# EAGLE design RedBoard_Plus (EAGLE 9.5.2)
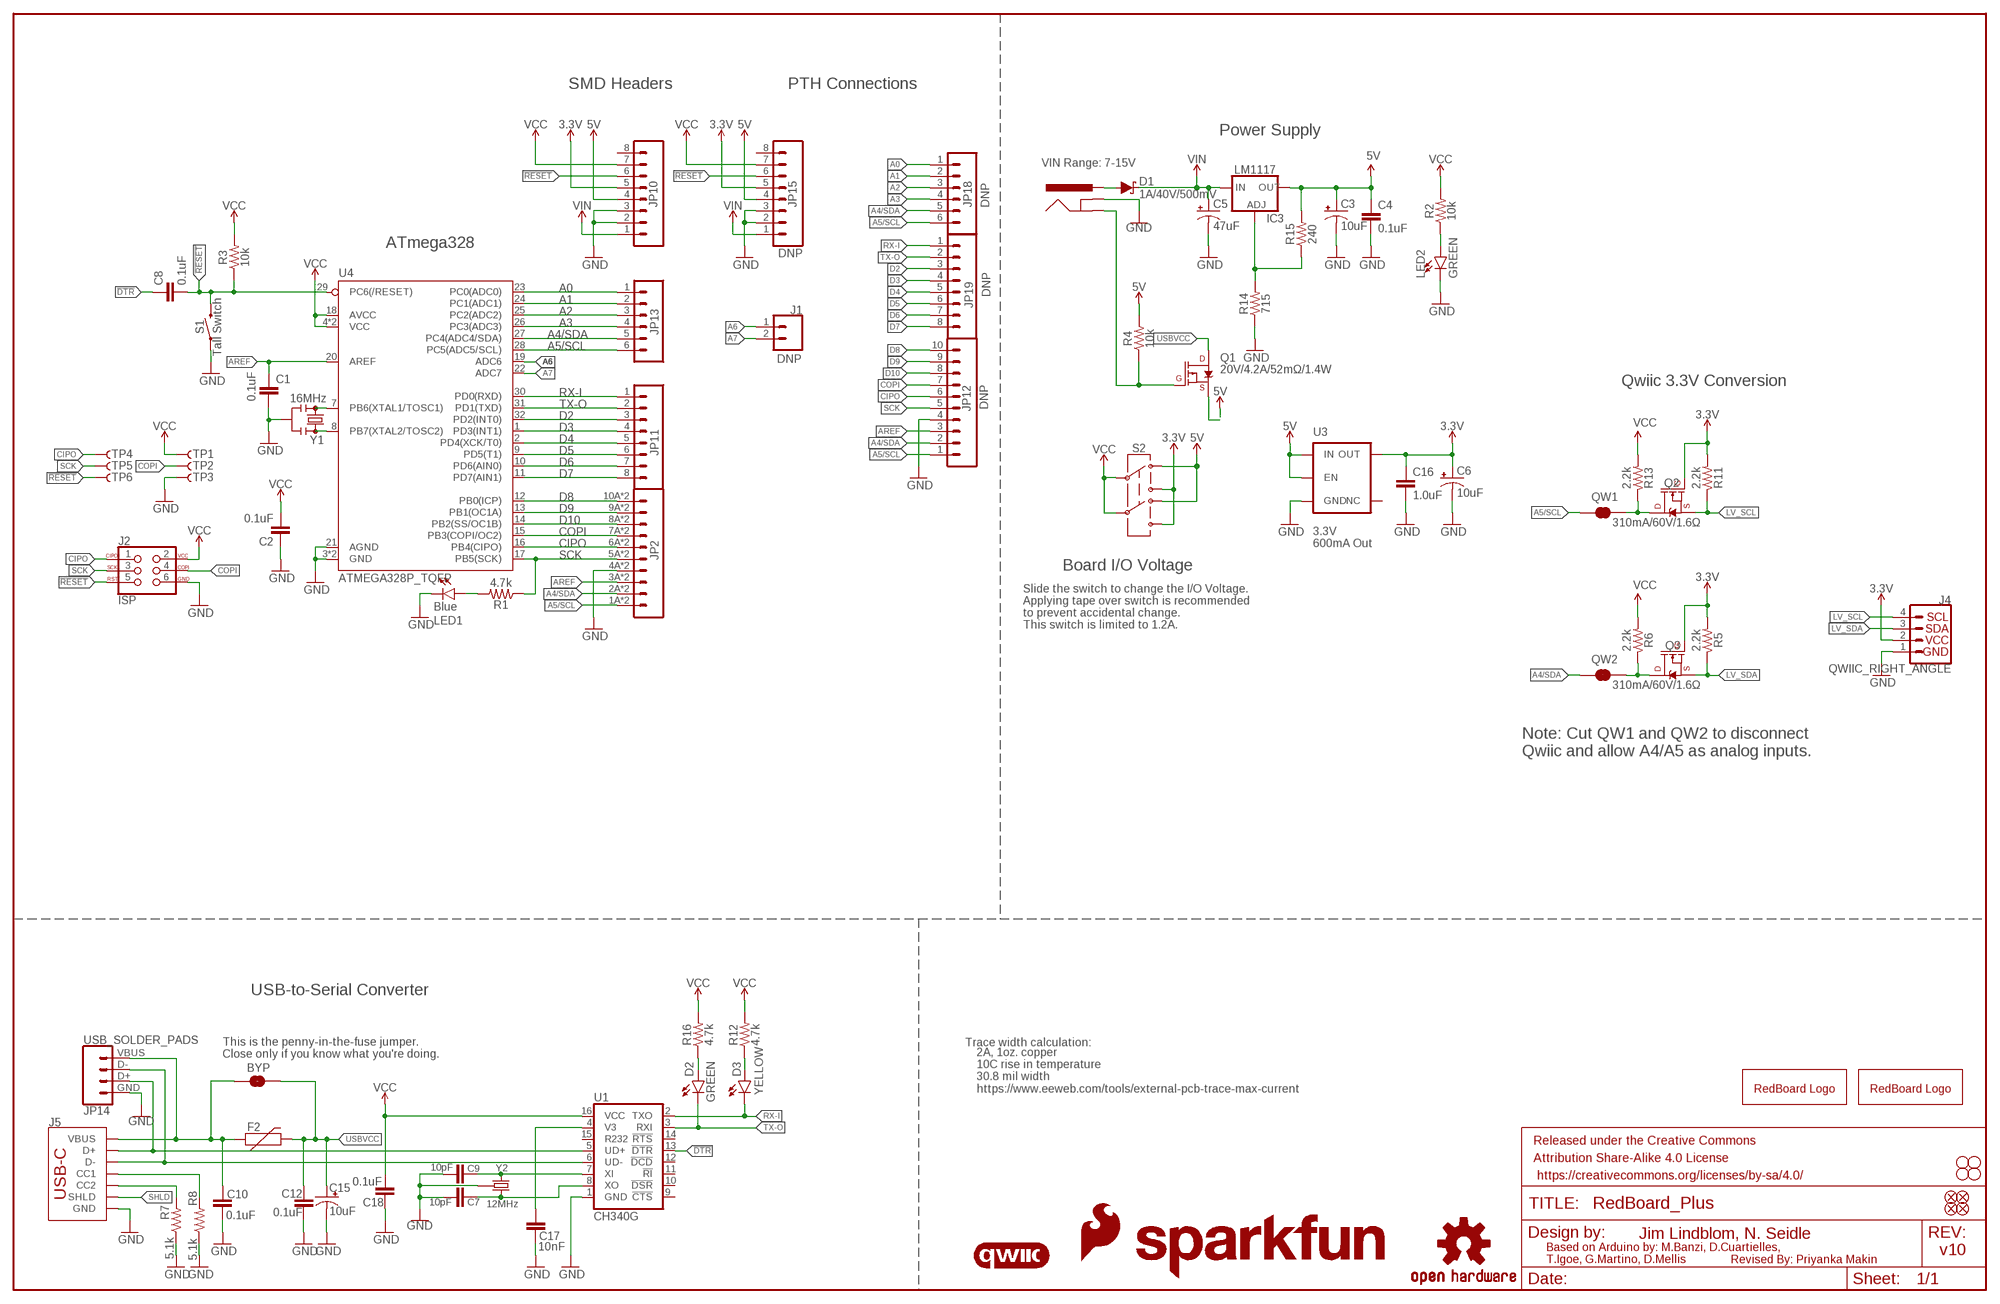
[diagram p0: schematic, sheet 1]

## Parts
BYP  JUMPER-SMT_2_NO_SILK  [SMT-JUMPER_2_NO_SILK]
C1  0.1uF  0.1UF-0603-25V-(+80/-20%)  [0603]
C2  0.1uF  0.1UF-0603-25V-(+80/-20%)  [0603]
C3  10uF  10UF-POLAR-EIA3216-16V-10%(TANT)  [EIA3216]
C4  0.1uF  0.1UF-0603-25V-(+80/-20%)  [0603]
C5  47uF  47UF-POLAR-PANASONIC_D-35V-20%  [PANASONIC_D]
C6  10uF  10UF-POLAR-EIA3216-16V-10%(TANT)  [EIA3216]
C7  10pF  10PF-0603-50V-5%  [0603]
C8  0.1uF  0.1UF-0603-25V-(+80/-20%)  [0603]
C9  10pF  10PF-0603-50V-5%  [0603]
C10  0.1uF  0.1UF-0603-25V-(+80/-20%)  [0603]
C12  0.1uF  0.1UF-0603-25V-(+80/-20%)  [0603]
C15  10uF  10UF-POLAR-EIA3216-16V-10%(TANT)  [EIA3216]
C16  1.0uF  1.0UF-0603-16V-10%  [0603]
C17  10nF  10NF-0603-50V-10%  [0603]
C18  0.1uF  0.1UF-0603-25V-(+80/-20%)  [0603]
D1  1A/40V/500mV  DIODE-SCHOTTKY-SS14  [SMA-DIODE]
D2  GREEN  LED-GREENLILYPAD  [LED-1206]
D3  YELLOW  LED-YELLOW_HIDDENSILK  [LED-1206-HIDDENSILK]
F2  6V/2A  PPTC_6V2A  [1210]
FD1  FIDUCIAL1X2  [FIDUCIAL-1X2]
FD2  FIDUCIAL1X2  [FIDUCIAL-1X2]
FRAME1  FRAME-LEDGER  [CREATIVE_COMMONS]
IC3  LM1117  V_REG_LM1117SOT223  [SOT223]
J1  DNP  CONN_021X02_NO_SILK  [1X02_NO_SILK]
J2  ISP  AVR_SPI_PROG_3X2SMD  [2X3_SMT_POSTS]
J3  5.5x2.1mm Barrel  POWER_JACKSMD  [POWER_JACK_SMD]
J4  QWIIC_RIGHT_ANGLE  QWIIC_CONNECTORJS-1MM  [JST04_1MM_RA]
J5  USB Female Type C Connector  USB_C_2-LAYER_PADS  [USB-C-16P-2LAYER-PADS]
JP1  SFE_LOGO_NAME.1_INCH  [SFE_LOGO_NAME_.1]
JP2  CONN_10SMD_COMBO-FEMALE  [1X10_SMD_COMBINED]
JP3  STAND-OFFTIGHT  [STAND-OFF-TIGHT]
JP4  STAND-OFFTIGHT  [STAND-OFF-TIGHT]
JP5  STAND-OFFTIGHT  [STAND-OFF-TIGHT]
JP6  STAND-OFFTIGHT  [STAND-OFF-TIGHT]
JP7  SFE_LOGO_FLAME.1_INCH  [SFE_LOGO_FLAME_.1]
JP8  FIDUCIAL1X2  [FIDUCIAL-1X2]
JP9  FIDUCIAL1X2  [FIDUCIAL-1X2]
JP10  CONN_08SMD-COMBO-FEMALE  [1X08_SMD_COMBINED]
JP11  JP11  CONN_08SMD-COMBO-FEMALE  [1X08_SMD_COMBINED]
JP12  DNP  CONN_10NO_SILK_PTH_FEMALE  [1X10_NO_SILK]
JP13  CONN_06SMD-STRAIGHT-COMBO-FEMALE  [1X06_SMD_STRAIGHT_COMBO]
JP14  USB_SOLDER_PADS  [USB-SOLDER-PADS]
JP15  DNP  CONN_08NO_SILK_DNP  [1X08_NO_SILK]
JP18  DNP  CONN_06NO_SILK_NO_POP  [1X06_NO_SILK]
JP19  DNP  CONN_08NO_SILK_DNP  [1X08_NO_SILK]
LED1  Blue  LED-BLUE_HIDDENSILK  [LED-1206-HIDDENSILK]
LED2  GREEN  LED-GREENLILYPAD  [LED-1206]
LOGO1  QWIIC_LOGO_5MM  [QWIIC_5MM]
Q1  20V/4.2A/52mΩ/1.4W  MOSFET_PCH-DMG2305UX-7  [SOT23-3]
Q2  310mA/60V/1.6Ω  MOSFET-NCH-2N7002PW  [SOT323]
Q3  310mA/60V/1.6Ω  MOSFET-NCH-2N7002PW  [SOT323]
QW1  JUMPER-SMT_2_NC_TRACE_SILK  [SMT-JUMPER_2_NC_TRACE_SILK]
QW2  JUMPER-SMT_2_NC_TRACE_SILK  [SMT-JUMPER_2_NC_TRACE_SILK]
R1  4.7k  4.7KOHM-0603-1/10W-1%  [0603]
R2  10k  10KOHM-0603-1/10W-1%  [0603]
R3  10k  10KOHM-0603-1/10W-1%  [0603]
R4  10k  10KOHM-0603-1/10W-1%  [0603]
R5  2.2k  2.2KOHM-0603-1/10W-1%  [0603]
R6  2.2k  2.2KOHM-0603-1/10W-1%  [0603]
R7  5.1k  5.1KOHM5.1KOHM-0603-1/10W-1%  [0603]
R8  5.1k  5.1KOHM5.1KOHM-0603-1/10W-1%  [0603]
R11  2.2k  2.2KOHM-0603-1/10W-1%  [0603]
R12  4.7k  4.7KOHM-0603-1/10W-1%  [0603]
R13  2.2k  2.2KOHM-0603-1/10W-1%  [0603]
R14  715  715OHM-0603-1/10W-1%  [0603]
R15  240  240OHM-0603-1/10W-1%  [0603]
R16  4.7k  4.7KOHM-0603-1/10W-1%  [0603]
S1  Tall Switch  MOMENTARY-SWITCH-SPST-SMD-5.2-TALL-REDUNDANT  [TACTILE_SWITCH_SMD_5.2MM]
S2  SWITCH-DPDT-SMD-AYZ0202  [SWITCH_DPDT_SMD_AYZ0202]
TP1  TP-3x5  TEST-POINT3X5  [PAD.03X.05]
TP2  TP-3x5  TEST-POINT3X5  [PAD.03X.05]
TP3  TP-3x5  TEST-POINT3X5  [PAD.03X.05]
TP4  TP-3x5  TEST-POINT3X5  [PAD.03X.05]
TP5  TP-3x5  TEST-POINT3X5  [PAD.03X.05]
TP6  TP-3x5  TEST-POINT3X5  [PAD.03X.05]
U1  CH340G  CH340GSMD  [SO016]
U3  3.3V  V_REG_AP2112K-3.3V  [SOT23-5]
U4  ATMEGA328P_TQFP  [TQFP32-08]
U$1  REDBOARD_LOGO  [REDBOARD_LOGO]
U$3  REDBOARD_LOGO  [REDBOARD_LOGO]
U$16  OSHW-LOGOS  [OSHW-LOGO-S]
Y1  16MHz  RESONATOR-16MHZSMD_3.2X1.3  [RESONATOR-SMD-3.2X1.3]
Y2  12MHz  CRYSTAL-GROUNDEDSMD-3.2X2.5  [CRYSTAL-SMD-3.2X2.5MM]

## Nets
3.3V [power]: C6.+ C16.1 J4.2 JP10.5 JP15.5 Q2.1(G) Q3.1(G) R5.2 R11.2 S2.1 S2.4 U3.5(OUT)
5V [power]: C3.+ C4.1 IC3.2(OUT) IC3.4(OUT) JP10.4 JP15.4 Q1.2(S) R4.2 R15.2 S2.3 S2.6 U3.1(IN) U3.3(EN)
!DTR!: C8.1 U1.13(!DTR)
!RESET: C8.2 J2.5 JP10.6 JP15.6 R3.1 S1.3 S1.4 TP6.P$1 U4.29(PC6(/RESET))
A0: JP13.1 JP18.1 U4.23(PC0(ADC0))
A1: JP13.2 JP18.2 U4.24(PC1(ADC1))
A2: JP13.3 JP18.3 U4.25(PC2(ADC2))
A3: JP13.4 JP18.4 U4.26(PC3(ADC3))
A4/SDA: JP2.2A JP2.2B JP12.2 JP13.5 JP18.5 QW2.1 U4.27(PC4(ADC4/SDA))
A5/SCL: JP2.1A JP2.1B JP12.1 JP13.6 JP18.6 QW1.1 U4.28(PC5(ADC5/SCL))
A6: J1.1 U4.19(ADC6)
A7: J1.2 U4.22(ADC7)
AREF: C1.1 JP2.3A JP2.3B JP12.3 U4.20(AREF)
CC1: J5.A5(CC1) R8.2
CC2: J5.B5(CC2) R7.2
CIPO: J2.1 JP2.6A JP2.6B JP12.6 TP4.P$1 U4.16(PB4(CIPO))
COPI: J2.4 JP2.7A JP2.7B JP12.7 TP2.P$1 U4.15(PB3(COPI/OC2))
D2: JP11.3 JP19.3 U4.32(PD2(INT0))
D3: JP11.4 JP19.4 U4.1(PD3(INT1))
D4: JP11.5 JP19.5 U4.2(PD4(XCK/T0))
D5: JP11.6 JP19.6 U4.9(PD5(T1))
D6: JP11.7 JP19.7 U4.10(PD6(AIN0))
D7: JP11.8 JP19.8 U4.11(PD7(AIN1))
D8: JP2.10A JP2.10B JP12.10 U4.12(PB0(ICP))
D9: JP2.9A JP2.9B JP12.9 U4.13(PB1(OC1A))
D10: JP2.8A JP2.8B JP12.8 U4.14(PB2(SS/OC1B))
D+: J5.A6(D+) J5.B6(D+) JP14.D+ U1.5(UD+)
D-: J5.A7(D-) J5.B7(D-) JP14.D- U1.6(UD-)
GND: C1.2 C2.1 C3.- C4.2 C5.- C6.- C7.2 C9.2 C10.2 C12.2 C15.- C16.2 C17.2 C18.2 J2.6 J3.GND(GNDBREAK) J4.1 J5.GND J5.GND2(GND) JP2.4A JP2.4B JP10.2 JP10.3 JP12.4 JP14.GND JP15.2 JP15.3 LED1.C LED2.C R7.1 R8.1 R14.1 S1.1 S1.2 TP3.P$1 U1.1(GND) U3.2(GND) U4.3(GND) U4.5(GND) U4.21(AGND) Y1.2 Y2.2(GND) Y2.4(GND)
INSERT: J3.P$4(GND) Q1.1(G) R4.1
LV_SCL: J4.4 Q2.2(S) R11.1
LV_SDA: J4.3 Q3.2(S) R5.1
N$1: LED1.A R1.2
N$2: LED2.A R2.1
N$3: U4.7(PB6(XTAL1/TOSC1)) Y1.1
N$4: U4.8(PB7(XTAL2/TOSC2)) Y1.3
N$5: D2.A R16.1
N$6: C17.1 U1.4(V3)
N$7: Q2.3(D) QW1.2 R13.1
N$8: C9.1 U1.7(XI) Y2.1
N$9: D3.A R12.1
N$10: C7.1 U1.8(XO) Y2.3
N$15: IC3.1(ADJ) R14.2 R15.1
N$45: Q3.3(D) QW2.2 R6.1
PWRIN [power]: D1.A J3.VIN0(PWR)
RX-I: D3.C JP11.1 JP19.1 U1.2(TXO) U4.30(PD0(RXD))
SCK: J2.3 JP2.5A JP2.5B JP12.5 R1.1 TP5.P$1 U4.17(PB5(SCK))
SHLD: J5.SHLD1(SHLD) J5.SHLD2(SHLD) J5.SHLD3(SHLD) J5.SHLD4(SHLD)
TX-O: D2.C JP11.2 JP19.2 U1.3(RXI) U4.31(PD1(TXD))
USBVCC [power]: BYP.2 C12.1 C15.+ F2.2 Q1.3(D)
VCC: C2.2 C18.1 J2.2 JP10.7 JP15.7 R2.2 R3.2 R6.2 R12.2 R13.2 R16.2 S2.2 S2.5 TP1.P$1 U1.16(VCC) U4.4(VCC) U4.6(VCC) U4.18(AVCC)
VIN [power]: C5.+ D1.C IC3.3(IN) JP10.1 JP15.1
VUSB [power]: BYP.1 C10.1 F2.1 J5.VBUS1(VBUS) J5.VBUS2(VBUS) JP14.VBUS
Unconnected: JP10.8 JP15.8 U1.9(!CTS) U1.10(!DSR) U1.11(!RI) U1.12(!DCD) U1.14(!RTS) U1.15(R232) U3.4(NC)

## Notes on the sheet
- SMD Headers | PTH Connections
- Power Supply
- VIN Range: 7-15V
- ATmega328
- Qwiic 3.3V Conversion
- 3.3V
  600mA Out
- Board I/O Voltage
- Slide the switch to change the I/O Voltage.
  Applying tape over switch is recommended
  to prevent accidental change.
- This switch is limited to 1.2A.
- Note: Cut QW1 and QW2 to disconnect 
  Qwiic and allow A4/A5 as analog inputs.
- USB-to-Serial Converter
- Trace width calculation:
- This is the penny-in-the-fuse jumper.
  Close only if you know what you're doing.
- 2A, 1oz. copper
  10C rise in temperature
  30.8 mil width
  https://www.eeweb.com/tools/external-pcb-trace-max-current
- Jim Lindblom, N. Seidle
- v10
- Based on Arduino by: M.Banzi, D.Cuartielles, 
  T.Igoe, G.Martino, D.Mellis
- Revised By: Priyanka Makin

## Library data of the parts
BYP = SparkFun-Jumpers:JUMPER-SMT_2_NO: Normally open jumper
C1 C2 C4 C8 C10 C12 C18 = SparkFun-Capacitors:0.1UF: 0.1µF ceramic capacitors; PROD_ID: CAP-00810
C3 C6 C15 = SparkFun-Capacitors:10UF-POLAR: 10.0µF polarized capacitors; PROD_ID: CAP-00811
C5 = SparkFun-Capacitors:47UF-POLAR: 47µF polarized capacitors; PROD_ID: CAP-08478
C7 C9 = SparkFun-Capacitors:10PF: 10pF ceramic capacitors; PROD_ID: CAP-11812
C16 = SparkFun-Capacitors:1.0UF: 1µF ceramic capacitors; PROD_ID: CAP-00868
C17 = SparkFun-Capacitors:10NF: 0.01uF/10nF/10,000pF ceramic capacitors; PROD_ID: CAP-00867
D1 = SparkFun-DiscreteSemi:DIODE-SCHOTTKY: Schottky diode; PROD_ID: DIO-08053
D2 LED2 = SparkFun-LED:LED-GREEN: Green SMD LED; PROD_ID: DIO-09910
D3 = SparkFun-LED:LED-YELLOW: Yellow SMD LED; PROD_ID: DIO-09909
F2 = SparkFun-Fuses:PPTC: Resettable Fuse PPTC; PROD_ID: RES-14313
FD1 FD2 JP8 JP9 = SparkFun-Aesthetics:FIDUCIAL: Fiducial Alignment Points
FRAME1 = SparkFun-Aesthetics:FRAME-LEDGER: Schematic Frame - Ledger
IC3 = SparkFun-IC-Power:V_REG_LM1117: Voltage Regulator LM1117 Standard adjustable voltage regulator but in SMD form. Spark Fun Electronics SKU : COM-00595; PROD_ID: VREG-08170
J1 = SparkFun-Connectors:CONN_02: Multi connection point. Often used as Generic Header-pin footprint for 0.1 inch spaced/style header connections
J2 = SparkFun-Connectors:AVR_SPI_PROG_3X2: AVR ISP 6 Pin This is the reduced ISP connector for AVR programming. Common on Arduino. This footprint will take up less PCB space and can be used with a 10-pin to 6-pin adapter such as SKU: BOB-08508 **Special note about "TEST_POINT" package. The stop mask is on the top side, so if you want your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; PROD_ID: CONN-11415
J3 = SparkFun-Connectors:POWER_JACK: Power Jack Connector This is the standard 5.5mm barrel jack for power. The PTH is the most common, proven, reliable, footprint. The Slot footprint only works if the mill layer is transmitted to the PCB fab house so be warned. Here are the connectors we sell at SparkFun: DC Barrel Power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; PROD_ID: CONN-08106; SF_ID: PRT-12748
J4 = SparkFun-Connectors:QWIIC_CONNECTOR: SparkFun I2C Standard Qwiic Connector An SMD 1mm pitch JST connector makes it easy and quick (get it? Qwiic?) to connect I2C devices to each other. The Qwiic system enables fast and solderless connection between popular platforms and various sensors and actuators. We carry 200mm, 100mm, 50mm, and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; PROD_ID: CONN-13694
J5 = SparkFun-Connectors:USB_C: USB Type C 16Pin Connector Super Speed pins not available on the 16-pin purely SMD connector so this part is best for USB 2.0 implementations. D1 and D2 are tied together enabling D+/- no matter which way the cable is plugged into the connector. The two channel configuration pins (CC1/2) are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; PROD_ID: CONN-14122
JP1 = SparkFun-Aesthetics:SFE_LOGO_NAME: SparkFun Font Logo
JP2 JP12 = SparkFun-Connectors:CONN_10: Multi connection point. Often used as Generic Header-pin footprint for 0.1 inch spaced/style header connections On any of the 0.1 inch spaced packages, you can populate with these: Break Away Headers - Straight (PRT-00116) Break Away Male Headers - Right Angle (PRT-00553) Female Headers (PRT-00115)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; PROD_ID: CONN-11219
JP3-JP6 = SparkFun-Hardware:STAND-OFF: Stand Off
JP7 = SparkFun-Aesthetics:SFE_LOGO_FLAME: SparkFun Flame Logo
JP10 JP11 = SparkFun-Connectors:CONN_08: Multi connection point. Often used as Generic Header-pin footprint for 0.1 inch spaced/style header connections On any of the 0.1 inch spaced packages, you can populate with these: Break Away Headers - Straight (PRT-00116) Break Away Male Headers - Right Angle (PRT-00553) Female Headers (PRT-00115)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; PROD_ID: CONN-10204; SF_ID: PRT-11543
JP13 JP18 = SparkFun-Connectors:CONN_06: Multi connection point. Often used as Generic Header-pin footprint for 0.1 inch spaced/style header connections On any of the 0.1 inch spaced packages, you can populate with these: Break Away Headers - Straight (PRT-00116) Break Away Male Headers - Right Angle (PRT-00553) Female Headers (PRT-00115)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; PROD_ID: CONN-10203
JP14 = SparkFun-Connectors:USB_SOLDER_PADS: Solder pad access to USB pins. Helpful to expose on PCBs so user can attach external USB connector if necessary.
JP15 = SparkFun-Connectors:CONN_08: Multi connection point. Often used as Generic Header-pin footprint for 0.1 inch spaced/style header connections On any of the 0.1 inch spaced packages, you can populate with these: Break Away Headers - Straight (PRT-00116) Break Away Male Headers - Right Angle (PRT-00553) Female Headers (PRT-00115)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; PROD_ID: CONN-10204
JP19 = SparkFun-Connectors:CONN_08: Multi connection point. Often used as Generic Header-pin footprint for 0.1 inch spaced/style header connections On any of the 0.1 inch spaced packages, you can populate with these: Break Away Headers - Straight (PRT-00116) Break Away Male Headers - Right Angle (PRT-00553) Female Headers (PRT-00115)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
LED1 = SparkFun-LED:LED-BLUE: Blue SMD LED; PROD_ID: DIO-09911
LOGO1 = SparkFun-Aesthetics:QWIIC_LOGO: Qwiic Logos for placement on schematic and PCB. The 5.5mm silk logo is best for placing next to Qwiic connector.
Q1 = SparkFun-DiscreteSemi:MOSFET_PCH: P-channel MOSFETs Voltage controlled devices that allow control of high current outputs. SparkFun Products: SparkFun ESP32 Thing SparkFun ESP8266 Thing SparkFun Pi Servo HAT V2 DMG2305UX-7 (20V/4.2A/SOT23-3); PROD_ID: TRANS-14388
Q2 Q3 = SparkFun-DiscreteSemi:MOSFET-NCH: N-channel MOSFETs Voltage controlled devices that allow control of high current outputs. SparkFun Products: SparkFun OpenScale SparkFun Digital Sandbox SparkFun Monster Moto Shield SparkFun MOSFET Power Controller; PROD_ID: TRANS-11151
QW1 QW2 = SparkFun-Jumpers:JUMPER-SMT_2_NC_TRACE: Normally closed trace jumper
R1 R12 R16 = SparkFun-Resistors:4.7KOHM: 4.7kΩ resistor; PROD_ID: RES-07857
R2-R4 = SparkFun-Resistors:10KOHM: 10kΩ resistor; PROD_ID: RES-00824
R5 R6 R11 R13 = SparkFun-Resistors:2.2KOHM: 2.2kΩ resistor; PROD_ID: RES-08272
R7 R8 = SparkFun-Resistors:5.1KOHM; PROD_ID: RES-12083
R14 = SparkFun-Resistors:715OHM: 715Ω resistor; PROD_ID: RES-07850
R15 = SparkFun-Resistors:240OHM: 240Ω resistor; PROD_ID: RES-07849
S1 = SparkFun-Switches:MOMENTARY-SWITCH-SPST: Momentary Switch (Pushbutton) - SPST; PROD_ID: SWCH-14139
S2 = SparkFun-Switches:SWITCH-DPDT: Double-Pole, Double-Throw (DPDT) Switch Double-pole, double-throw switches. Variant Overview PTH-GPI-152-3013 Used on SparkFun Geiger Counter SMD-AY0202 Surface Mount DPDT Switch (COM-00597) Used on e.g. LilyPad Arduino USB - ATmega32U4 Board; PROD_ID: SWCH-08179; SF_SKU: COM-00597
TP1-TP6 = SparkFun-Connectors:TEST-POINT: SparkFun Test Points
U1 = SparkFun-IC-Comms:CH340G: A simple USB 2.0 to Serial IC.; PROD_ID: IC-13498
U3 = SparkFun-IC-Power:V_REG_AP2112: AP2112 - 600mA CMOS LDO Regulator w/ Enable The AP2112 is CMOS process low dropout linear regulator with enable function, the regulator delivers a guaranteed 600mA (min.) continuous load current. Features Output Voltage Accuracy: ±1.5% Output Current: 600mA (Min.) Foldback Short Current Protection: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; PROD_ID: VREG-12457
U4 = SparkFun-IC-Microcontroller:ATMEGA328P_TQFP: Popular 328P in QFP Storefront component: ATmega328 - TQFP (COM-13448) Datasheet SparkFun Products SparkFun RedBoard - Programmed with Arduino (DEV-12757) Arduino Pro Mini 328 - 5V/16MHz (DEV-11113) Arduino Pro Mini 328 - 3.3V/8MHz (DEV-11114) SparkFun OpenLog (DEV-13712) SparkFun MicroView - OLED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; PROD_ID: IC-09069
U$1 U$3 = SparkFun-Aesthetics:REDBOARD_LOGO
U$16 = SparkFun-Aesthetics:OSHW-LOGO: Open-Source Hardware (OSHW) Logo
Y1 = SparkFun-Clocks:RESONATOR-16MHZ: 16MHz Resonator Digikey Example Frequency: 16MHz Frequency Stability: &plusmn;0.3% Frequency Tolerance: &plusmn;0.5% Capacitance: 15pF SparkFun Products SparkFun OpenLog SparkFun MicroView - OLED Arduino Module; PROD_ID: XTAL-08900
Y2 = SparkFun-Clocks:CRYSTAL-GROUNDED: Crystals w/ Ground Pin (Generic) These are passive quartz crystals, which can be used as a clock source for a microcontroller. Crystal's are usually two-terminal devices. A third terminal may be optionally connected to ground, as recommended by the manufaturer.; PROD_ID: XTAL-13518

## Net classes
0 default: width 0 mm, drill 0 mm
1 power: width 0.762 mm

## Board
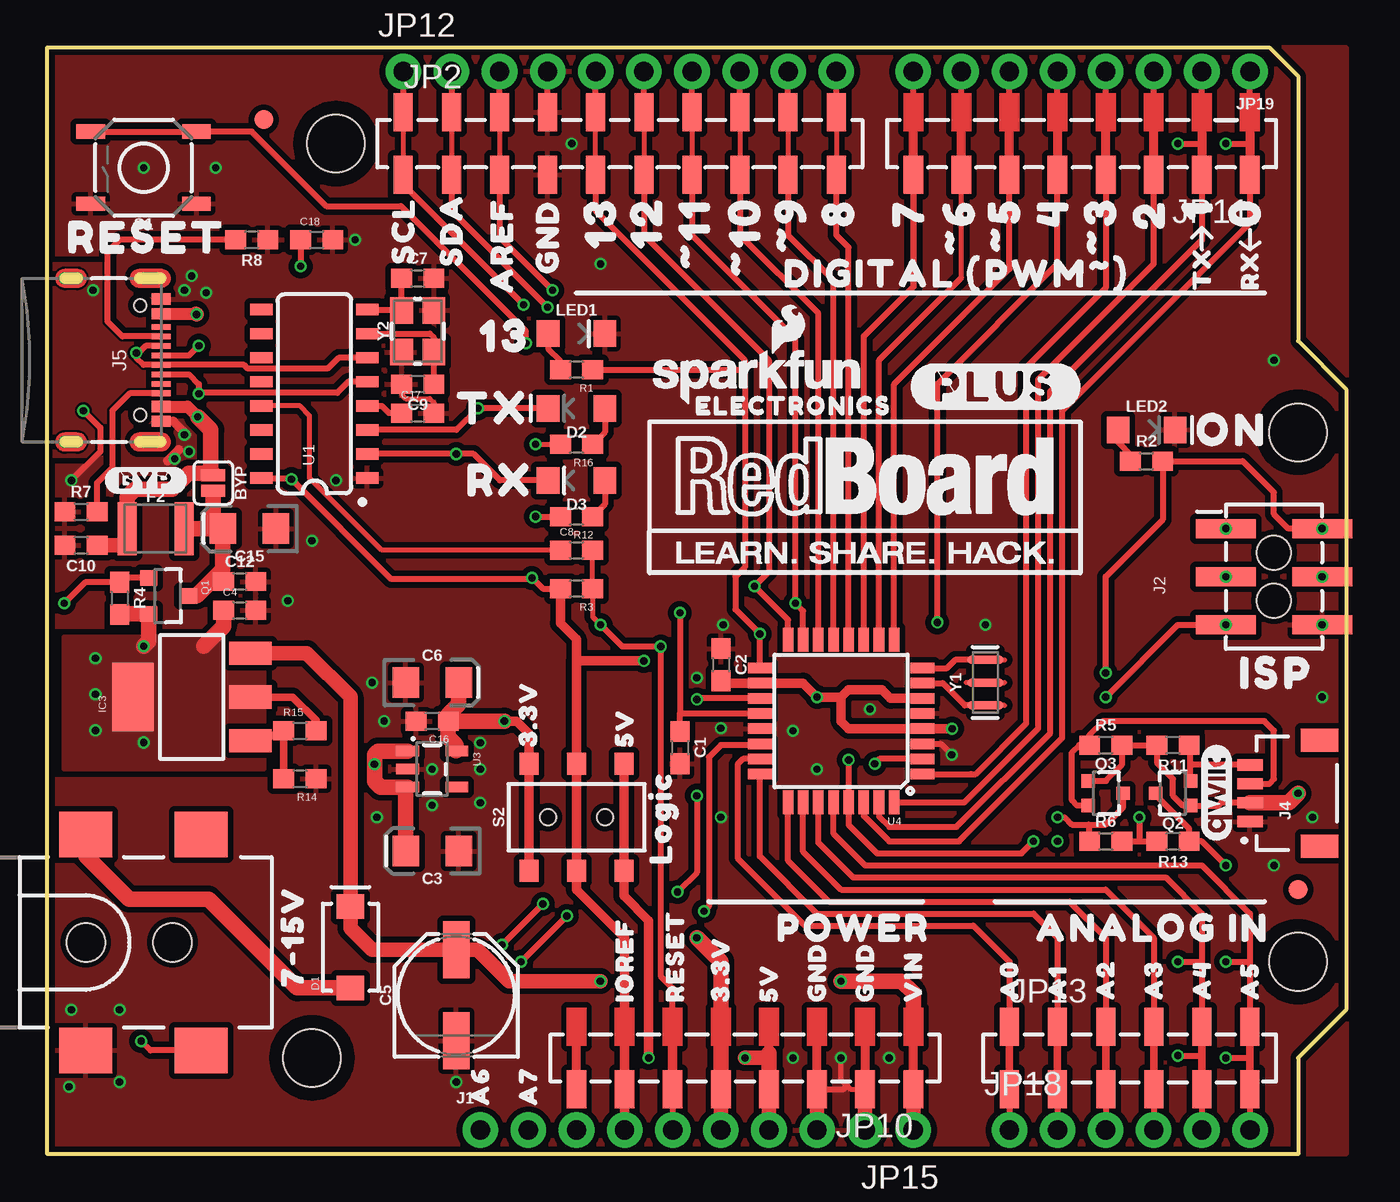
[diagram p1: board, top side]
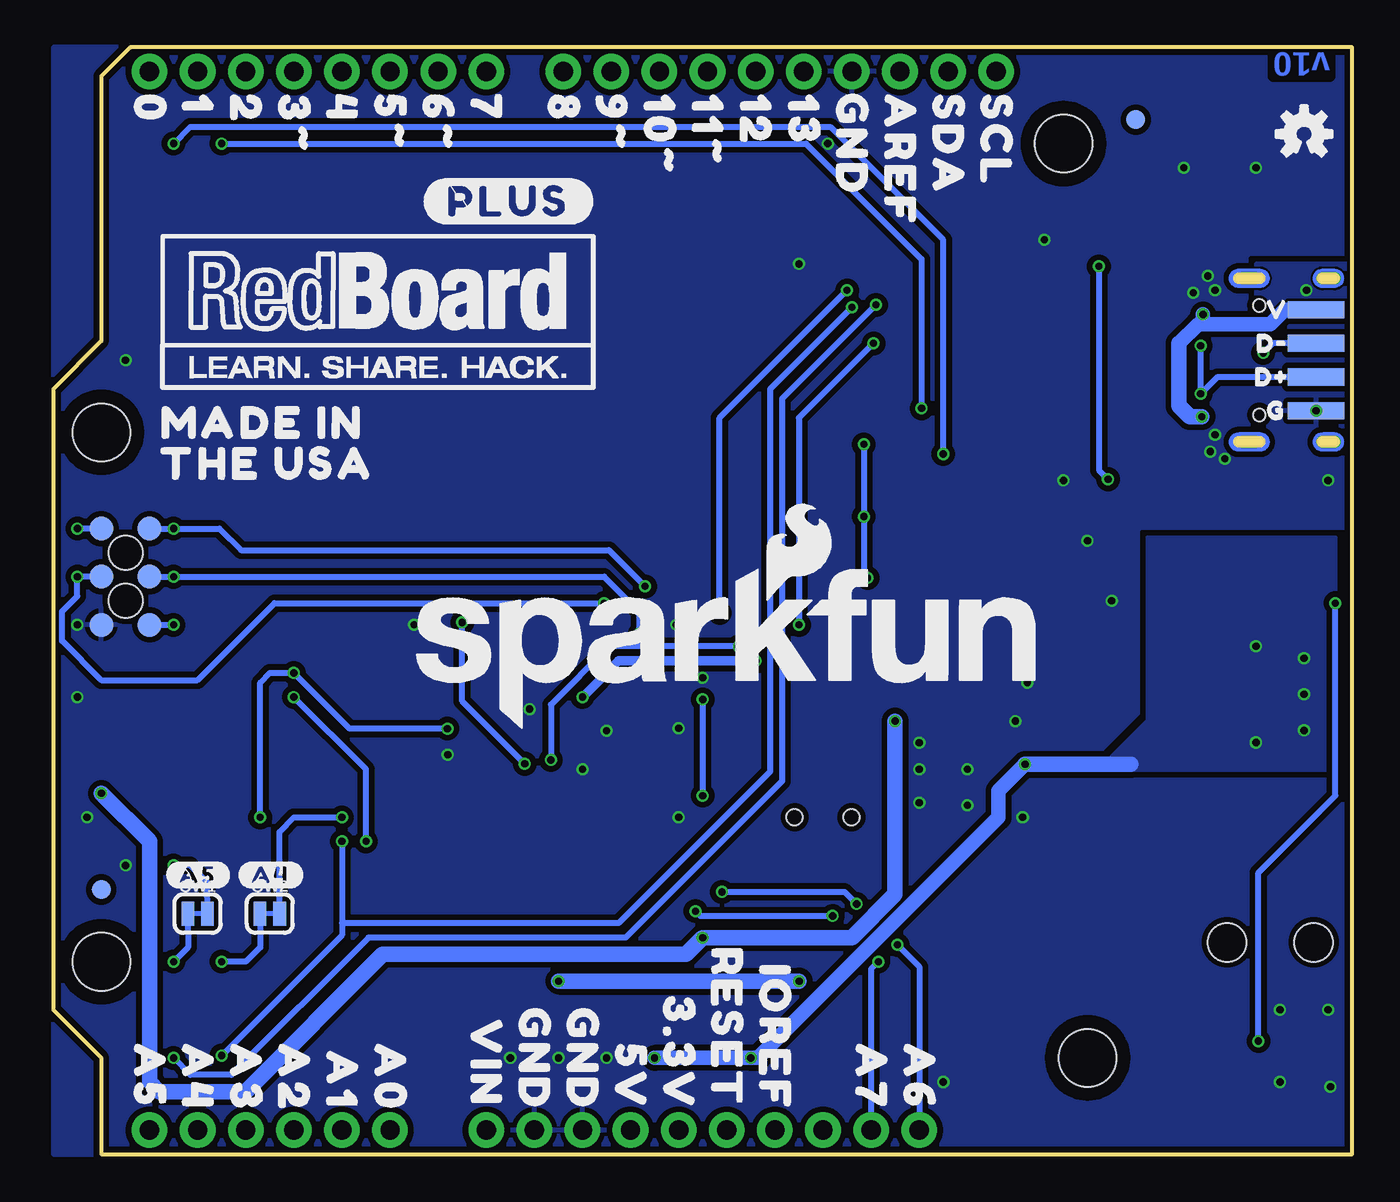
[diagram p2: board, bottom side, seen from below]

Size 68.58 x 58.42 mm. Coordinates in mm from the lower left corner, seen from the top.
Outline: 0,58.42 64.52,58.42 66.04,56.9 66.04,42.93 68.58,40.39 68.58,7.62 66.04,5.08 66.04,0 0,0 0,58.42
Copper layers (1*16): Top 0.035mm / dielectric 1.5mm / Bottom 0.035mm
Design rules "SparkFun-2-Layer-Minimum-JLCPCB": minimum track width 5mil, minimum drill 0.3mm, track to track 5mil, track to pad 5mil, pad to pad 5mil, via to via 5mil, smd to smd 5mil, copper to edge 7mil, drill to drill 7mil, minimum pad ring 5mil, minimum via ring 5mil, stop-mask expansion 2.5mil, vias tented up to drill 25mil, thermal gap 10mil
vRestrict: area 0.6,22.4 to 2,30.6; area 5.7,23.1 to 7.4,30.6; area 47.9,10.8 to 48.5,11.3; area 50.4,10.7 to 50.9,11.6; area 11.3,29.3 to 12.7,31.6; area 0.3,13 to 9.4,25

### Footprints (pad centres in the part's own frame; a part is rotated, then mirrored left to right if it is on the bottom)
SMT-JUMPER_2_NO_SILK = smd 0.635 x 1.27: 1 -0.406,0; 2 0.406,0
0603 = smd 1.1 x 1: 1 -0.85,0; 2 0.85,0
EIA3216 = smd 1.4 x 1.6: + 1.4,0; - -1.4,0
PANASONIC_D = smd 3 x 1.4: + 2.4,0; - -2.4,0
SMA-DIODE = smd 1.27 x 1.47: A -2.15,0; C 2.15,0
LED-1206 = smd 1.2 x 1.4: A -1.5,0; C 1.5,0
LED-1206-HIDDENSILK = smd 1.2 x 1.4: A -1.5,0; C 1.5,0
1210 = smd 1 x 2.8: 1 -1.5,0; 2 1.5,0
FIDUCIAL-1X2 = smd 1 x 1: 1 0,0
SOT223 = smd 1.219 x 2.235: 1 -2.311,-3.099; 2 0,-3.099; 3 2.311,-3.099 | smd 3.6 x 2.2: 4 0,3.099
1X02_NO_SILK = drill 1.016 pad 1.88: 1 0,0; 2 2.54,0
2X3_SMT_POSTS = smd 1 x 3.17: 1 -2.54,-2.54; 2 -2.54,2.54; 3 0,-2.54; 4 0,2.54; 5 2.54,-2.54; 6 2.54,2.54 | hole 1.8: -1.27,0; 1.27,0
POWER_JACK_SMD = smd 2.8 x 2.4: GND 0,-5.7; P$4 6.1,-5.7; VIN0 0,5.7; VIN1 6.1,5.7 | hole 2.032: 0,0; 4.572,0
JST04_1MM_RA = smd 0.6 x 1.35: 1 -1.5,0; 2 -0.5,0; 3 0.5,0; 4 1.5,0 | smd 1.2 x 2: NC1 2.8,-3.675; NC2 -2.8,-3.675
USB-C-16P-2LAYER-PADS = smd 0.3 x 1: A5 -1.25,-0.34; A6 -0.25,-0.34; A7 0.25,-0.34; A8 1.25,-0.34; B5 1.75,-0.34; B6 0.75,-0.34; B7 -0.75,-0.34; B8 -1.75,-0.34 | smd 0.6 x 1: GND -3.225,-0.34; GND2 3.225,-0.34; VBUS1 -2.45,-0.34; VBUS2 2.45,-0.34 | drill 0.4 pad 0.6 long: SHLD1 -4.318,-0.915; SHLD2 4.318,-0.915; SHLD3 -4.318,-5.095; SHLD4 4.318,-5.095 | hole 0.65: -2.89,-1.445; 2.89,-1.445
1X10_SMD_COMBINED = smd 1 x 2: 1A 0,1.65; 1B 0,-1.65; 2A 2.54,1.65; 2B 2.54,-1.65; 3A 5.08,1.65; 3B 5.08,-1.65; 4A 7.62,1.65; 4B 7.62,-1.65; 5A 10.16,1.65; 5B 10.16,-1.65; 6A 12.7,1.65; 6B 12.7,-1.65; 7A 15.24,1.65; 7B 15.24,-1.65; 8A 17.78,1.65; 8B 17.78,-1.65; 9A 20.32,1.65; 9B 20.32,-1.65; 10A 22.86,1.65; 10B 22.86,-1.65
STAND-OFF-TIGHT = hole 3.048: 0,0
1X08_SMD_COMBINED = smd 1 x 2: 1 0,1.65; 2 2.54,1.65; 3 5.08,1.65; 4 7.62,1.652; 5 10.16,1.65; 6 12.7,1.652; 7 15.24,1.65; 8 17.78,1.652
1X10_NO_SILK = drill 1.016 pad 1.88: 1 0,0; 2 2.54,0; 3 5.08,0; 4 7.62,0; 5 10.16,0; 6 12.7,0; 7 15.24,0; 8 17.78,0; 9 20.32,0; 10 22.86,0
1X06_SMD_STRAIGHT_COMBO = smd 1 x 2: 1 0,-1.65; 1-2 0,1.65; 2 2.54,1.65; 2-2 2.54,-1.65; 3 5.08,-1.65; 3-2 5.08,1.65; 4 7.62,1.65; 4-2 7.62,-1.65; 5 10.16,-1.65; 5-2 10.16,1.65; 6 12.7,1.65; 6-2 12.7,-1.65
USB-SOLDER-PADS = smd 3 x 0.9: D+ 0,-0.889; D- 0,0.889; GND 0,-2.667; VBUS 0,2.667
1X08_NO_SILK = drill 1.016 pad 1.88: 1 0,0; 2 2.54,0; 3 5.08,0; 4 7.62,0; 5 10.16,0; 6 12.7,0; 7 15.24,0; 8 17.78,0
1X06_NO_SILK = drill 1.016 pad 1.88: 1 0,0; 2 2.54,0; 3 5.08,0; 4 7.62,0; 5 10.16,0; 6 12.7,0
SOT23-3 = smd 0.8 x 0.9: 1 -0.95,-1; 2 0.95,-1; 3 0,1.1
SOT323 = smd 0.7 x 0.7: 1 -0.65,-0.925; 2 0.65,-0.925; 3 0,0.925
SMT-JUMPER_2_NC_TRACE_SILK = smd 0.66 x 1.27: 1 -0.521,0; 2 0.521,0
TACTILE_SWITCH_SMD_5.2MM = smd 1.524 x 0.762: 1 -2.794,1.905; 2 2.794,1.905; 3 -2.794,-1.905; 4 2.794,-1.905
SWITCH_DPDT_SMD_AYZ0202 = smd 1 x 1.15: 1 -2.5,2.825; 2 0,2.825; 3 2.5,2.825; 4 -2.5,-2.825; 5 0,-2.825; 6 2.5,-2.825 | hole 0.85: 1.5,0; -1.5,0
PAD.03X.05 = smd 1.27 x 1.27: P$1 0,0
SO016 = smd 0.6 x 1.2: 1 -4.445,-2.8; 2 -3.175,-2.8; 3 -1.905,-2.8; 4 -0.635,-2.8; 5 0.635,-2.8; 6 1.905,-2.8; 7 3.175,-2.8; 8 4.445,-2.8; 9 4.445,2.8; 10 3.175,2.8; 11 1.905,2.8; 12 0.635,2.8; 13 -0.635,2.8; 14 -1.905,2.8; 15 -3.175,2.8; 16 -4.445,2.8
SOT23-5 = smd 0.55 x 1.2: 1 -0.95,-1.3; 2 0,-1.3; 3 0.95,-1.3; 4 0.95,1.3; 5 -0.95,1.3
TQFP32-08 = smd 1.27 x 0.559: 1 -4.293,2.8; 2 -4.293,2; 3 -4.293,1.2; 4 -4.293,0.4; 5 -4.293,-0.4; 6 -4.293,-1.2; 7 -4.293,-2; 8 -4.293,-2.8; 17 4.293,-2.8; 18 4.293,-2; 19 4.293,-1.2; 20 4.293,-0.4; 21 4.293,0.4; 22 4.293,1.2; 23 4.293,2; 24 4.293,2.8 | smd 0.559 x 1.27: 9 -2.8,-4.293; 10 -2,-4.293; 11 -1.2,-4.293; 12 -0.4,-4.293; 13 0.4,-4.293; 14 1.2,-4.293; 15 2,-4.293; 16 2.8,-4.293; 25 2.8,4.293; 26 2,4.293; 27 1.2,4.293; 28 0.4,4.293; 29 -0.4,4.293; 30 -1.2,4.293; 31 -2,4.293; 32 -2.8,4.293
RESONATOR-SMD-3.2X1.3 = smd 0.45 x 1.905: 1 -1.2,0; 2 0,0; 3 1.2,0
CRYSTAL-SMD-3.2X2.5MM = smd 1.4 x 1.2: 1 -1.1,-0.85; 2 1.1,-0.85; 3 1.1,0.85; 4 -1.1,0.85

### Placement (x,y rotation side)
BYP  8.76,35.43 270 top
C1  33.4,21.46 270 top
C2  35.56,25.84 270 top
C3  20.32,16 180 top
C4  10.16,28.7 0 top
C5  21.59,8.38 90 top
C6  20.32,24.89 0 top
C7  19.56,46.23 0 top
C8  27.94,31.88 0 top
C9  19.56,40.64 180 top
C10  1.78,32.13 180 top
C12  10.16,30.23 0 top
C15  10.67,33.02 180 top
C16  20.32,22.86 180 top
C17  19.56,39.12 0 top
C18  14.22,48.26 0 top
D1  16,10.92 90 top
D2  27.94,39.37 180 top
D3  27.94,35.56 180 top
F2  5.71,33.02 0 top
FD1  11.43,54.61 0 bottom
FD2  66.04,13.97 0 bottom
FRAME1  not placed on the board
IC3  7.62,24.13 90 top
J1  22.86,1.27 0 top
J2  64.77,30.48 270 top
J3  2.03,11.18 0 top
J4  63.5,19.05 90 top
J5  6.35,41.91 270 top
JP1  37.47,41.02 0 top
JP2  18.8,53.34 0 top
JP3  13.97,5.08 0 top
JP4  66.04,10.16 0 top
JP5  66.04,38.1 0 top
JP6  15.24,53.34 0 top
JP7  39.12,43.56 0 top
JP8  66.04,13.97 0 top
JP9  11.43,54.61 0 top
JP10  45.72,5.08 180 top
JP11  63.5,53.34 180 top
JP12  18.8,57.15 0 top
JP13  50.8,5.08 0 top
JP14  1.91,41.91 0 bottom
JP15  45.72,1.27 180 top
JP18  50.8,1.27 0 top
JP19  63.5,57.15 180 top
LED1  27.94,43.31 0 top
LED2  58.04,38.23 0 top
LOGO1  61.72,19.05 90 top
Q1  6.35,29.46 270 top
Q2  59.44,19.05 90 top
Q3  55.88,19.05 270 top
QW1  60.96,12.7 0 bottom
QW2  57.15,12.7 0 bottom
R1  27.94,41.4 180 top
R2  58.04,36.58 0 top
R3  27.94,29.84 180 top
R4  3.81,29.34 270 top
R5  55.88,21.59 0 top
R6  55.88,16.51 0 top
R7  1.78,33.91 0 top
R8  10.79,48.26 180 top
R11  59.44,21.59 180 top
R12  27.94,33.66 180 top
R13  59.44,16.51 180 top
R14  13.34,19.81 180 top
R15  13.34,22.35 0 top
R16  27.94,37.47 180 top
S1  5.08,52.07 180 top
S2  27.94,17.78 0 top
TP1  66.04,33.02 0 bottom
TP2  66.04,30.48 0 bottom
TP3  66.04,27.94 0 bottom
TP4  63.5,33.02 0 bottom
TP5  63.5,30.48 0 bottom
TP6  63.5,27.94 0 bottom
U1  14.1,40.13 90 top
U3  20.32,20.32 270 top
U4  41.91,22.86 180 top
U$1  31.75,30.48 0 top
U$2  [_D#0]  6.1,42.8 0 bottom
U$3  62.87,40.26 0 bottom
U$4  [V0]  5.21,44.58 0 bottom
U$9  [10#0]  36.58,57.15 270 bottom
U$10  [G0]  5.21,39.24 0 bottom
U$11  [LOGIC0]  32.38,14.48 90 top
U$12  [D#0]  5.84,41.02 0 bottom
U$13  [_RESET0]  -0.76,48.39 0 top
U$14  [#BYP#0]  3.05,35.56 0 top
U$16  2.54,53.85 0 bottom
U$17  [7#15V0]  12.95,8 90 top
U$18  [_AREF0]  24,44.2 90 top
U$19  [_SCL0]  18.8,45.72 90 top
U$20  [_SDA0]  21.34,45.59 90 top
U$21  [11#0]  34.04,57.15 270 bottom
U$22  [130]  29.21,46.61 90 top
U$23  [120]  31.62,46.61 90 top
U$24  [#110]  34.16,45.47 90 top
U$25  [#100]  36.83,45.09 90 top
U$26  [#90]  39.24,46.35 90 top
U$27  [80]  41.78,47.75 90 top
U$28  [70]  45.47,47.75 90 top
U$29  [#60]  48.13,46.23 90 top
U$30  [#50]  50.55,46.35 90 top
U$31  [40]  53.09,47.75 90 top
U$32  [#30]  55.63,46.23 90 top
U$33  [20]  58.17,47.62 90 top
U$34  [10]  60.71,48.13 90 top
U$35  [00]  63.25,47.75 90 top
U$36  [TX0]  60.96,44.96 90 top
U$37  [RX0]  63.5,44.96 90 top
U$38  [DIGITAL_##PWM####_0]  37.85,46.48 0 top
U$39  [13_0]  21.59,43.18 0 top
U$40  [_TX0]  19.81,39.37 0 top
U$41  [_RX0]  20.32,35.56 0 top
U$42  [_GND0]  26.42,45.21 90 top
U$43  [3#3V0]  25.4,20.83 90 top
U$44  [5V0]  30.48,20.83 90 top
U$45  [ON0]  59.44,38.23 0 top
U$46  [ISP0]  61.72,25.4 0 top
U$47  [POWER0]  37.47,11.94 0 top
U$48  [ANALOG_IN0]  51.18,11.94 0 top
U$49  [IOREF0]  30.48,7.37 90 top
U$50  [RESET0]  33.15,7.37 90 top
U$51  [3#3V0]  35.56,7.37 90 top
U$52  [5V0]  38.1,7.37 90 top
U$53  [GND0]  40.64,7.37 90 top
U$54  [GND0]  43.18,7.37 90 top
U$55  [VIN0]  45.72,7.37 90 top
U$56  [A00]  50.8,7.49 90 top
U$57  [A10]  53.34,7.49 90 top
U$58  [A20]  55.88,7.49 90 top
U$59  [A30]  58.42,7.49 90 top
U$60  [A40]  60.96,7.49 90 top
U$61  [A50]  63.5,7.49 90 top
U$62  [A60]  22.86,1.91 90 top
U$63  [A70]  25.4,1.91 90 top
U$64  [00]  63.5,57.15 270 bottom
U$65  [10]  60.96,57.15 270 bottom
U$66  [20]  58.42,57.15 270 bottom
U$67  [3#0]  55.88,57.15 270 bottom
U$68  [40]  53.34,57.15 270 bottom
U$69  [5#0]  50.8,57.15 270 bottom
U$70  [6#0]  48.26,57.15 270 bottom
U$71  [70]  45.72,57.15 270 bottom
U$72  [80]  41.66,57.15 270 bottom
U$73  [9#0]  39.12,57.15 270 bottom
U$76  [120]  31.5,57.15 270 bottom
U$77  [130]  28.96,57.15 270 bottom
U$78  [SFE_LOGO_NAME_.3]  33.02,26.67 0 bottom
U$79  [AREF0]  23.88,57.15 270 bottom
U$80  [SDA0]  21.34,57.15 270 bottom
U$81  [SCL0]  18.8,57.15 270 bottom
U$82  [MADE_IN0]  64.14,38.61 0 bottom
U$83  [THE_USA0]  64.14,36.45 0 bottom
U$84  [_A40]  60.96,7.62 270 bottom
U$85  [_GND_0]  26.42,57.78 270 bottom
U$86  [_A30]  58.42,7.62 270 bottom
U$87  [_A20]  55.88,7.62 270 bottom
U$88  [_A10]  53.34,7.24 270 bottom
U$89  [_A00]  50.8,7.62 270 bottom
U$90  [_VIN0]  45.72,8.89 270 bottom
U$93  [_5V0]  38.1,7.62 270 bottom
U$94  [_3#3V0]  35.56,10.16 270 bottom
U$95  [_RESET0]  33.02,12.7 270 bottom
U$96  [_IOREF0]  30.48,11.81 270 bottom
U$97  [_A60]  22.86,7.62 270 bottom
U$98  [_A70]  25.4,7.62 270 bottom
U$99  [_GND_0]  40.64,9.53 270 bottom
U$100  [#PLUS#0]  45.59,40.51 0 top
U$101  [SFE_LOGO_FLAME_.2]  29.21,31.75 0 bottom
U$102  [_A50]  63.5,7.62 270 bottom
U$103  [#PLUS#0]  49.02,50.29 0 bottom
U$104  [ELECTRONICS0]  33.53,39.5 0 top
U$105  [#A4#0]  58.8,14.73 0 bottom
U$106  [#A5#0]  62.61,14.73 0 bottom
U$107  [_GND_0]  43.18,9.53 270 bottom
Y1  49.53,24.89 90 top
Y2  19.56,43.43 90 top

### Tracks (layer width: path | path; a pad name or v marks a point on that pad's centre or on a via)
3.3V  (via drill 0.38)
  Top 0.305: J4.2 61.98,18.55 61.83,18.4 Q2.1 59.96,18.4 59.44,18.92 59.44,19.81 58.59,20.66 R11.2 R5.2 56.73,20.54 55.9,19.7 Q3.1
  Top 0.508: 21.59,21.3 U3.5 | v24.13,22.86 24.77,22.86 25.44,22.18 S2.1 S2.4
  Top 0.762: JP10.5 JP15.5
  Top 0.813: JP10.5 35.56,10.16 v34.29,11.43 | C6.+ 21.72,23.75 21.17,23.2 C16.1 | C16.1 v24.13,22.86 | C16.1 21.17,22.01 21.59,21.59 21.59,21.3 | J4.2 65.54,18.55 v66.04,19.05
  Bottom 0.813: v24.13,22.86 24.13,13.72 26.42,11.43 v34.29,11.43 35.18,10.54 51.18,10.54 58.42,3.3 62.99,3.3 63.5,3.81 63.5,16.51 v66.04,19.05
5V  (via drill 0.38)
  Top 0.406: IC3.2 12.95,24.13 14.19,22.9 R15.2
  Top 0.508: 18.92,19.27 U3.3 | v31.75,5.08 31.75,12.32 30.44,13.63 S2.6 S2.3
  Top 0.762: v36.83,5.08 37.85,5.08 38.1,5.33 | JP10.4 JP15.4
  Top 0.813: JP10.4 38.1,5.33 38.1,4.57 JP10.4 | C3.+ 18.92,19.27 | v5.08,26.81 5.35,27.08 Q1.2 3.84,28.51 R4.2 | U3.3 17.59,19.37 17.27,19.68 v17.27,20.57 17.27,21.08 17.46,21.27 U3.1 | C4.1 9.31,27.85 8.26,26.8
  Bottom 0.762: v36.83,5.08 v31.75,5.08 31.37,5.08 18.67,17.78 18.67,19.18 v17.27,20.57
  Bottom 0.813: v17.27,20.57 11.68,20.57
  other vias: 2.54,24.27 5.08,21.73 2.54,22.36 2.54,26.17
  pour Bottom (isolate 0.305, no thermals): 0.89,32.51 10.79,32.51 10.79,22.86 12.7,20.95 12.7,20.32 0.89,20.32
  pour Top (isolate 0.305, no thermals): 0.89,20.32 0.89,27.3 11.43,27.3 11.43,20.32
!DTR!
  Top 0.254: C8.1 25.4,31.88 25.27,31.88 17.65,31.88 13.84,35.69 13.84,38.99 13.34,39.5 U1.13
!RESET  (via drill 0.38, 0.38 pad 0.51)
  Top 0.254: C8.2 R3.1 28.79,28.36 v29.21,27.94
  Top 0.305: v42.31,20.81 U4.29 42.31,17.38 43.81,15.88 51.44,15.88 v52.07,16.51 | v29.21,27.94 30.35,26.8 v32.38,26.8 32.38,9.4 33.02,8.76 JP10.6 JP15.6 | v25.27,42.8 25.27,43.43 18.67,50.04 14.73,50.04 10.79,53.98 S1.3 S1.4 | v55.88,24.13 59.69,27.94 J2.5
  Bottom 0.305: v42.31,20.81 42.31,23.73 39.24,26.8 v32.38,26.8 | v29.21,27.94 29.21,38.86 v25.27,42.8 | v52.07,16.51 52.07,20.32 v55.88,24.13 | TP6.P$1 J2.5
  other vias: 62.23,27.94
A0
  Top 0.305: U4.23 36.73,20.86 36.45,20.57 36.45,15.62 40.01,12.06 48.9,12.06 50.8,10.16 JP13.1 JP18.1
A1
  Top 0.254: JP13.2 53.34,3.43
  Top 0.305: U4.24 37.62,15.72 40.64,12.7 52.07,12.7 53.34,11.43 JP13.2 | 53.34,3.43 JP18.2
A2
  Top 0.305: U4.25 39.11,15.5 41.27,13.34 53.98,13.34 55.88,11.43 55.88,3.81 JP13.3 JP18.3
A3
  Top 0.254: JP13.4 58.42,3.43
  Top 0.305: U4.26 39.91,15.97 41.91,13.97 55.88,13.97 58.42,11.43 JP13.4 | 58.42,3.43 JP18.4
A4/SDA  (via drill 0.38)
  Top 0.254: JP2.2A JP2.2B
  Top 0.305: U4.27 40.71,16.44 42.55,14.61 59.05,14.61 60.96,12.7 60.96,10.16 | 60.96,10.16 60.96,5.21 | 60.96,5.21 JP13.5 JP18.5 | JP2.2B 21.34,49.78 v26.42,44.7 | v59.69,5.21 60.96,5.21 | v59.69,10.16 60.96,10.16 | JP12.2 JP2.2A
  Bottom 0.305: 53.34,12.19 38.73,12.19 30.73,20.19 30.73,40.39 v26.42,44.7 | v59.69,5.21 53.34,11.56 53.34,12.19 | v53.34,16.51 53.34,12.19 | QW2.1 57.66,10.92 58.42,10.16 v59.69,10.16
A5/SCL  (via drill 0.38)
  Top 0.254: 63.5,5.08 63.5,3.43 | JP2.1A 18.8,54.61 JP2.1B
  Top 0.305: U4.28 41.51,16.91 43.18,15.24 60.96,15.24 63.5,12.7 63.5,10.16 | 63.5,10.16 JP13.6 63.5,5.08 v62.23,5.08 | JP2.1B 19.05,51.44 19.05,50.93 v25.15,44.83 | v62.23,10.16 63.5,10.16 | JP12.1 18.8,54.61 | 63.5,3.43 JP18.6
  Bottom 0.305: v25.15,44.83 30.1,39.88 30.1,19.68 38.35,11.43 51.94,11.43 59.18,4.19 61.34,4.19 v62.23,5.08 | QW1.1 61.47,10.92 v62.23,10.16
A6  (via drill 0.38)
  Top 0.305: v34.29,24 34.35,24.06 U4.19 | v34.29,18.92 34.29,14.86 v33.27,13.84 | v26.16,13.21 v24,11.05
  Bottom 0.305: v34.29,24 v34.29,18.92 | v33.27,13.84 26.8,13.84 v26.16,13.21 | v24,11.05 22.86,9.91 J1.1
A7  (via drill 0.38)
  Top 0.305: U4.22 37.55,21.59 35.56,21.59 34.92,20.95 34.92,13.08 v34.67,12.83 | v27.43,12.57 v25.02,10.16
  Bottom 0.305: v34.67,12.83 34.42,12.57 v27.43,12.57 | v25.02,10.16 25.4,9.78 J1.2
AREF  (via drill 0.38)
  Top 0.254: JP2.3A JP2.3B
  Top 0.305: 33.4,23.26 U4.20 | v33.4,28.57 33.4,23.26 | C1.1 33.4,23.26 | JP2.3B 23.88,48.39 v26.67,45.59 | JP2.3A JP12.3
  Bottom 0.305: v26.67,45.59 33.4,38.86 v33.4,28.57
CC1
  Top 0.305: J5.A5 3.96,43.16 3.17,43.94 3.17,47.62 3.81,48.26 R8.2
CC2
  Top 0.305: J5.B5 4.35,40.16 3.43,39.24 3.43,36.23 2.63,35.43 R7.2
CIPO  (via drill 0.38, 0.38 pad 0.51)
  Top 0.254: JP2.6A JP2.6B
  Top 0.305: U4.16 39.11,28.2 v37.34,29.97 38.1,30.73 38.1,41.91 31.5,48.51 JP2.6B | JP2.6A JP12.6
  Bottom 0.305: v37.34,29.97 39.24,31.88 58.67,31.88 59.82,33.02 J2.1 TP4.P$1
  other vias: 62.23,33.02
COPI  (via drill 0.38, 0.38 pad 0.51)
  Top 0.254: JP2.7A JP2.7B
  Top 0.305: U4.15 39.91,28.67 v39.5,29.08 39.5,43.05 34.04,48.51 JP2.7B | JP2.7A JP12.7
  Bottom 0.305: v39.5,29.08 56.9,29.08 60.96,25.02 66.04,25.02 68.11,27.09 68.11,28.65 67.31,29.45 J2.4 TP2.P$1
  other vias: 67.31,30.48
D2
  Top 0.254: 58.42,54.99 JP11.3
  Top 0.305: JP11.3 58.42,46.99 52.32,40.89 52.32,22.48 48.41,18.57 U4.32 | 58.42,54.99 JP19.3
D3
  Top 0.254: JP11.4 55.88,52.07
  Top 0.305: 55.88,52.07 55.88,50.8 55.88,45.72 51.69,41.53 51.69,22.73 49.02,20.07 48.77,20.07 48.76,20.06 U4.1 | JP11.4 JP19.4
D4  (via drill 0.38)
  Top 0.254: 53.34,54.99 JP11.5
  Top 0.305: v46.99,28.07 46.99,40.64 53.34,46.99 JP11.5 | U4.2 43.94,20.86 v43.69,20.61 | 53.34,54.99 JP19.5
  Bottom 0.305: v43.69,20.61 46.99,23.91 v46.99,28.07
D5
  Top 0.254: JP11.6
  Top 0.305: U4.9 44.71,40.64 50.8,46.73 JP11.6 | JP11.6 JP19.6
D6
  Top 0.254: 48.26,46.26 JP11.7 48.26,54.99
  Top 0.305: U4.10 43.91,41.91 48.26,46.26 | 48.26,54.99 JP19.7
D7
  Top 0.254: JP11.8 45.72,52.07
  Top 0.305: U4.11 43.11,43.18 45.72,45.79 | JP11.8 JP19.8
  Top 0.356: 45.72,52.07 45.72,45.79
D8
  Top 0.254: JP2.10A JP2.10B
  Top 0.305: U4.12 42.31,47.86 41.66,48.51 JP2.10B | JP2.10A JP12.10
D9
  Top 0.254: JP2.9A JP2.9B
  Top 0.305: U4.13 41.51,46.12 39.12,48.51 JP2.9B | JP2.9A JP12.9
D10
  Top 0.254: JP2.8A JP2.8B
  Top 0.305: U4.14 40.71,44.38 36.58,48.51 JP2.8B | JP2.8A JP12.8
D+  (via drill 0.38)
  Top 0.305: J5.B6 7.48,41.16 8,40.64 v8,40.13 8.06,40.19 15.3,40.19 15.88,40.77 U1.5 | v8,42.67 7.49,42.16 J5.A6
  Bottom 0.305: v8,42.67 v8,40.13 7.11,41.02 JP14.D+
D-  (via drill 0.38)
  Top 0.305: J5.B7 5.2,42.66 4.83,42.29 v4.7,42.29 4.7,42.04 5.08,41.66 J5.A7 10.38,41.66 10.58,41.46 14.79,41.46 15.37,42.04 U1.6
  Bottom 0.305: JP14.D- 4.19,42.8 v4.7,42.29
GND  (via drill 0.38, 0.38 pad 0.51)
  Top 0.254: JP10.2 42.42,3.43 42.23,3.62 41.91,3.94 v41.91,5.08 | C9.2 18.71,40.09 18.92,39.88 20.19,39.88 20.41,39.66 C17.2
  Top 0.305: U4.3 47.17,21.66 v47.75,21.08 | JP10.3 42.04,3.43 42.23,3.62 | JP2.4A JP12.4 | JP14.GND 2.79,38.35 2.79,37.08 v1.27,35.56
  Top 0.508: 6.94,37.19 6.35,36.6 | 6.65,38.69 7.37,37.97
  Top 0.762: JP10.2 JP15.2 | JP10.3 JP15.3
  other vias: 5.08,52.07 64.77,41.91 40.64,20.32 27.69,53.34 43.43,23.5 49.53,27.94 35.69,27.94 1.27,7.62 29.21,46.99 67.31,24.13 17.78,22.86 17.4,17.78 67.31,27.94 6.73,36.7 13.97,32.38 15.24,35.56 12.7,29.21 8.89,52.07 35.56,17.78 39.37,22.35 7.62,46.35 20.32,20.32 22.86,20.32 22.86,21.72 22.86,18.54 20.32,18.41 17.14,24.89 16.26,48.26 3.81,3.81 3.81,7.62 1.14,3.56 21.59,3.81 64.77,15.24 66.8,17.78 44.45,5.08 39.37,5.08 35.56,22.48 34.29,25.15 1.91,39.24 7.24,37.97 7.49,37.08 7.24,45.59 8.38,45.47
  pour Top (isolate 0.305, rank 2): 0,58.42 68.58,58.42 68.58,0 0,0
  pour Bottom (isolate 0.305, rank 2): 0,58.42 68.58,58.42 68.58,0 0,0
INSERT  (via drill 0.38)
  Top 0.305: J3.P$4 5.45,5.48 v4.95,5.97 | Q1.1 4.04,30.41 R4.1 1.99,30.19 v0.89,29.08
  Bottom 0.305: v4.95,5.97 4.95,14.86 0.89,18.92 v0.89,29.08
LV_SCL
  Top 0.305: Q2.2 60.36,20.57 | 60.36,20.57 60.36,21.52 R11.1 | J4.4 60.38,20.55 60.36,20.57
LV_SDA
  Top 0.305: J4.3 64.51,19.55 64.77,19.81 64.77,22.35 64.26,22.86 55.75,22.86 55.03,22.14 R5.1 54.48,21.59 54.1,21.21 54.1,18.67 54.37,18.4 Q3.2
N$1
  Top 0.305: R1.2 27.09,41.87 26.44,42.52 LED1.A
N$2
  Top 0.356: R2.1 57.19,36.92 56.54,37.57 LED2.A
N$3
  Top 0.305: U4.7 47.28,24.86 48.44,23.69 Y1.1
N$4
  Top 0.305: U4.8 47.5,25.66 47.94,26.09 Y1.3
N$5
  Top 0.305: D2.A 29.44,38.12 R16.1
N$6
  Top 0.305: U1.4 17.66,39.5 18.04,39.12 C17.1
N$7  (via drill 0.38)
  Top 0.305: Q2.3 58.59,18.98 58.59,18.88 60.29,17.18 R13.1 60.96,16.51 v62.23,15.24
  Bottom 0.305: QW1.2 60.45,14.35 61.34,15.24 v62.23,15.24
N$8
  Top 0.305: U1.7 17.99,43.31 20.19,43.31 20.41,43.09 Y2.1 C9.1
N$9
  Top 0.305: D3.A 29.44,34.3 R12.1
N$10
  Top 0.305: U1.8 18.66,44.58 Y2.3 C7.1
N$15
  Top 0.305: IC3.1 11.61,21.82 12.14,22.35 R15.1
  Top 0.406: R14.2 R15.1
N$45  (via drill 0.38)
  Top 0.254: 55.03,17.36 54.99,17.4
  Top 0.305: v53.34,17.78 53.72,17.78 54.1,17.4 54.99,17.4 55.88,17.4 56.8,18.32 Q3.3 | R6.1 55.03,17.36
  Bottom 0.305: QW2.2 56.64,17.02 55.88,17.78 v53.34,17.78
PWRIN
  Top 0.813: J3.VIN0 2.03,15.75 4.32,13.46 8.51,13.46 13.2,8.77 D1.A
RX-I  (via drill 0.38)
  Top 0.254: 63.5,54.99 63.5,52.07
  Top 0.305: U4.30 43.11,17.85 44.45,16.51 48.13,16.51 53.59,21.97 53.59,39.24 63.5,49.15 JP11.1 63.5,52.07 63.5,53.34 v62.23,53.34 | 63.5,54.99 JP19.1 | D3.C 23.9,35.56 22.5,36.96 v21.59,36.96 U1.2
  Bottom 0.305: v21.59,36.96 21.59,48.26 27.56,54.23 61.34,54.23 v62.23,53.34
SCK  (via drill 0.38, 0.38 pad 0.51)
  Top 0.254: JP2.5B JP2.5A
  Top 0.305: U4.17 v37.62,27.46 36.32,28.75 36.32,30.48 36.83,30.99 36.83,41.4 | JP2.5B 28.96,49.78 36.83,41.91 36.83,41.4 | R1.1 36.83,41.4 | JP2.5A JP12.5
  Bottom 0.305: v37.62,27.46 37.62,28.6 39.5,30.48 J2.3 TP5.P$1
  other vias: 62.23,30.48
SHLD  (via drill 0.38)
  other vias: 2.41,45.59
  pour Bottom: 0,46.99 5.08,46.99 5.08,36.83 0,36.83
  pour Top: 0,46.99 5.08,46.99 5.08,36.83 0,36.83
TX-O  (via drill 0.38)
  Top 0.305: U4.31 43.91,17.81 44.45,17.27 48.01,17.27 52.96,22.23 52.96,40.26 60.96,48.26 JP11.2 | v59.69,53.34 60.96,53.34 JP11.2 | JP11.2 JP19.2 | D2.C v22.73,39.37 21.59,38.23 U1.3
  Bottom 0.305: v22.73,39.37 22.73,47.24 28.83,53.34 v59.69,53.34
USBVCC
  Top 0.254: BYP.2 8.76,34.82
  Top 0.813: F2.2 C15.+ | C15.+ 8.76,33.52 8.76,34.82 | Q1.3 7.87,29.46 8.64,30.23 | 8.64,30.23 C12.1 | C15.+ 9.27,30.86 8.64,30.23
VCC  (via drill 0.38)
  Top 0.254: v25.78,37.47 R16.2
  Top 0.305: v55.88,25.4 55.88,30.48 58.89,33.49 R2.2 63.12,36.58 64.77,34.92 64.77,33.78 65.53,33.02 J2.2 | R3.2 26.16,29.84 v25.59,30.42 25.53,30.35 18.16,30.35 v12.89,35.62 12.83,35.69 U1.16 | R6.2 57.66,16.51 | 57.66,16.51 R13.2 | v57.66,17.78 57.66,16.51 | C18.1 v13.37,46.86 | v25.78,33.66 R12.2
  Top 0.508: U4.6 44.52,24.06 44.07,24.51 42.29,24.51 41.91,24.13 | C2.2 35.69,24.86 U4.18 39.91,24.86 v40.64,24.13 41.91,24.13 | v47.77,22.46 U4.4 42.31,22.46 41.91,22.86 41.91,24.13 | v31.5,26.04 27.94,26.04 | R3.2 27.09,28.03 27.94,27.18 27.94,26.04 | 27.94,26.04 S2.2 S2.5 27.94,13.97 30.48,11.43 JP10.7 JP15.7
  Bottom 0.305: v47.77,22.46 52.94,22.46 v55.88,25.4 57.15,25.4 57.66,24.89 v57.66,17.78 | v25.78,37.47 v25.78,33.66 25.78,30.61 v25.59,30.42 | TP1.P$1 J2.2 | v13.37,46.86 13.37,36.11 v12.89,35.62
  Bottom 0.508: v40.64,24.13 38.73,26.04 v31.5,26.04
  other vias: 67.31,33.02
VIN  (via drill 0.38)
  Top 0.305: JP10.1 45.72,6.73
  Top 0.762: v29.2,9.13 24.38,9.13 22.73,10.78 C5.+ 17.16,10.78 16,11.94 D1.C 16,24.14 13.7,26.44 IC3.3 | JP10.1 JP15.1
  Top 0.813: v41.9,9.13 45.1,9.13 45.72,8.51 45.72,6.73
  Bottom 0.813: v41.9,9.13 v29.2,9.13
VUSB  (via drill 0.38)
  Top 0.254: 8.76,35.94 BYP.1 8.64,35.97
  Top 0.635: J5.VBUS2 7.4,39.46 v7.94,38.92 | J5.VBUS1 7.84,44.36
  Top 0.762: 7.84,44.36 v7.87,44.32 | C10.1 4.19,32.13 4.19,33 F2.1
  Top 0.813: F2.1 4.21,34.7 4.61,35.09 6.6,35.09 7.46,35.94 8.76,35.94 | v7.94,38.92 8.64,38.23 8.64,35.97
  Bottom 0.762: JP14.VBUS 3.56,44.58 4.32,43.81 7.87,43.81 | 9.14,42.8 8.13,43.81 7.87,43.81 | v7.87,44.32 7.87,43.81
  Bottom 0.813: 9.14,42.8 9.14,39.5 8.57,38.92 v7.94,38.92

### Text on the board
Bottom: v10
Measures: Units in inches
tDocu: Jim Lindblom / N. Seidle | Revised By: Priyanka Makin | Based on Arduino by: M.Banzi, D.Cuartielles, / T.Igoe, G.Martino, D.Mellis
214bmp: D:/SmartProjects/Snc/a4_bn_logo2.bmp

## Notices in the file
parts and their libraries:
SparkFun-Aesthetics: Licensing: CC v3.0 Share-Alike You are welcome to use this library for commercial purposes.
SparkFun-Aesthetics: Released under the Creative Commons Attribution Share-Alike 4.0 License
SparkFun-Aesthetics: https://creativecommons.org/licenses/by-sa/4.0
